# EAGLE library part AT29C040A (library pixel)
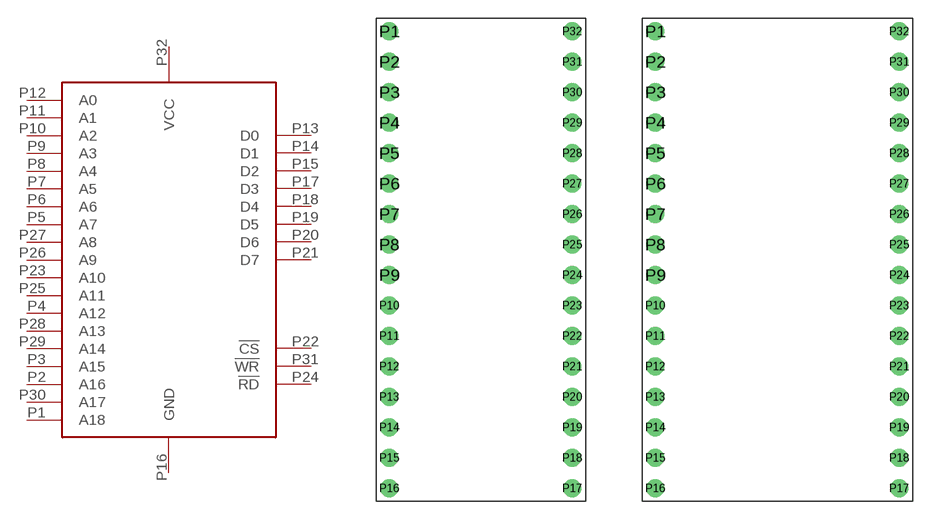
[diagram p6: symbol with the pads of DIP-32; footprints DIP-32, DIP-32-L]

Designator prefix -

## AT29C040A  [DIP-32]
P1  A18
P2  A16
P3  A15
P4  A12
P5  A7
P6  A6
P7  A5
P8  A4
P9  A3
P10  A2
P11  A1
P12  A0
P13  D0
P14  D1
P15  D2
P16  GND
P17  D3
P18  D4
P19  D5
P20  D6
P21  D7
P22  !CS
P23  A10
P24  !RD
P25  A11
P26  A9
P27  A8
P28  A13
P29  A14
P30  A17
P31  !WR
P32  VCC

## AT29C040ALARGE  [DIP-32-L]
Pads as for DIP-32

## Footprint DIP-32 (pad centres in mm)
drill 1.016: P1 -7.62,19.05; P2 -7.62,16.51; P3 -7.62,13.97; P4 -7.62,11.43; P5 -7.62,8.89; P6 -7.62,6.35; P7 -7.62,3.81; P8 -7.62,1.27; P9 -7.62,-1.27; P10 -7.62,-3.81; P11 -7.62,-6.35; P12 -7.62,-8.89; P13 -7.62,-11.43; P14 -7.62,-13.97; P15 -7.62,-16.51; P16 -7.62,-19.05; P17 7.62,-19.05; P18 7.62,-16.51; P19 7.62,-13.97; P20 7.62,-11.43; P21 7.62,-8.89; P22 7.62,-6.35; P23 7.62,-3.81; P24 7.62,-1.27; P25 7.62,1.27; P26 7.62,3.81; P27 7.62,6.35; P28 7.62,8.89; P29 7.62,11.43; P30 7.62,13.97; P31 7.62,16.51; P32 7.62,19.05

## Footprint DIP-32-L (pad centres in mm)
drill 1.016: P1 -10.16,19.05; P2 -10.16,16.51; P3 -10.16,13.97; P4 -10.16,11.43; P5 -10.16,8.89; P6 -10.16,6.35; P7 -10.16,3.81; P8 -10.16,1.27; P9 -10.16,-1.27; P10 -10.16,-3.81; P11 -10.16,-6.35; P12 -10.16,-8.89; P13 -10.16,-11.43; P14 -10.16,-13.97; P15 -10.16,-16.51; P16 -10.16,-19.05; P17 10.16,-19.05; P18 10.16,-16.51; P19 10.16,-13.97; P20 10.16,-11.43; P21 10.16,-8.89; P22 10.16,-6.35; P23 10.16,-3.81; P24 10.16,-1.27; P25 10.16,1.27; P26 10.16,3.81; P27 10.16,6.35; P28 10.16,8.89; P29 10.16,11.43; P30 10.16,13.97; P31 10.16,16.51; P32 10.16,19.05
